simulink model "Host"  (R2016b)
settings: Solver=ode45  StartTime=0.0  StopTime=inf  RelTol=1e-3  AbsTol=1e-6
PreLoadFcn:
  | % load standard fuelsys data
  | load targets_fsysdat;
  | % load standard definitions for the failure signals
  | targets_fsysdat_failsigs;
undefined symbols (not defined in the file or in its folder): period, rep_seq_t, rep_seq_y, serial
libraries: dspnetwork x5, etargetslib x2, instrumentlib x2, demo_controls x1, simulink_extras x1

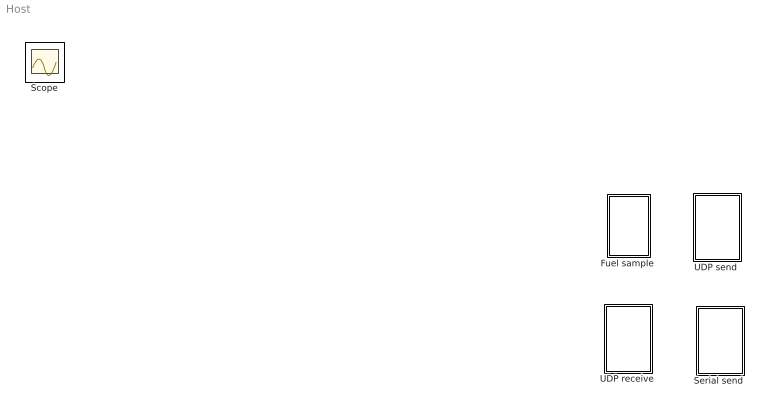
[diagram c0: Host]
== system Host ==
  "Fuel sample " : Subsystem  Commented=on
  "Serial send " : Subsystem  Commented=on
  "UDP receive " : Subsystem
  "UDP send " : Subsystem  Commented=on
  Scope : Scope

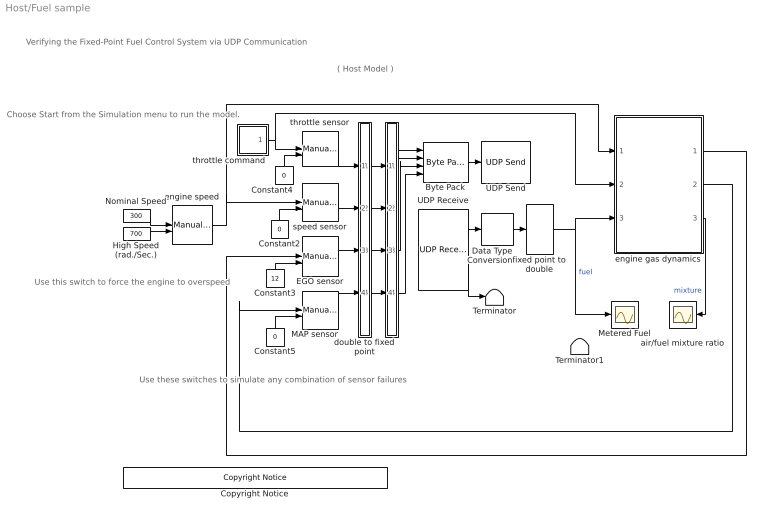
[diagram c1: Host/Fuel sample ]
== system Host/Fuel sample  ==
  note: Use these switches to simulate any combination of sensor failures
  note: Use this switch to force the engine to overspeed
  note: Choose Start from the Simulation menu to run the model.
  note: Verifying the Fixed-Point Fuel Control System via UDP Communication
  note: ( Host Model )
  " " : Subsystem
  Byte Pack : etargetslib/Byte Pack  datatypes={'uint16', 'uint16', 'uint16', 'uint16'}  byteAlign=1
  Constant2 : Constant  Value=0
  Constant3 : Constant  Value=12
  Constant4 : Constant  Value=0
  Constant5 : Constant  Value=0
  Copyright Notice : demo_controls/Copyright Notice  year=2015  prod=idelink
  Data Type Conversion : DataTypeConversion  OutDataTypeStr=fixdt(1,16,8)  ConvertRealWorld=Stored Integer (SI)
  EGO sensor : ManualSwitch
  High Speed (rad./Sec.) : Constant  Value=700
  MAP sensor : ManualSwitch  CurrentSetting=0
  Metered Fuel : Scope
  Nominal Speed : Constant  Value=300
  Terminator : Terminator
  Terminator1 : Terminator
  UDP Receive : dspnetwork/UDP Receive  localURL='0.0.0.0'  localPort=25000  remoteURL='0.0.0.0'  remotePort=-1  recvBufferSize=8192  dims=1  signalDatatype=uint16  isVarSize=off  showBlockingTime=on  blockingTime=1  sampletime=0.01  blockPlatform=HOST
  UDP Send : dspnetwork/UDP Send  remoteURL='255.255.255.255'  remotePort=25555  localURL='255.255.255.255'  localPortSource=Automatically determine  localPort=-1  sampletime=-1  blockPlatform=HOST  separateLengthPort=0
  air/fuel mixture ratio : Scope
  double to fixed point : Subsystem
  engine speed : ManualSwitch
  engine gas dynamics : Subsystem
  fixed point to double : DataTypeConversion  OutDataTypeStr=double  SampleTime=0
  speed sensor : ManualSwitch
  throttle command : Subsystem
  throttle sensor : ManualSwitch
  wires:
  double to fixed point/4(Out4) -> " "/4(In4)
  double to fixed point/1(Out1) -> " "/1(In1)
  double to fixed point/3(Out3) -> " "/3(In3)
  double to fixed point/2(Out2) -> " "/2(In2)
  UDP Receive/2 -> Terminator/1
  Data Type Conversion/1 -> fixed point to double/1
  MAP sensor/1 -> double to fixed point/4(In4)
  engine gas dynamics/3(air/fuel ratio) -> air/fuel mixture ratio/1  "mixture"
  speed sensor/1 -> double to fixed point/2(In2)
  throttle sensor/1 -> double to fixed point/1(In1)
  engine gas dynamics/1(o2_out) -> EGO sensor/1
  engine speed/1 -> engine gas dynamics/1(engine speed), speed sensor/1
  EGO sensor/1 -> double to fixed point/3(In3)
  Constant5/1 -> MAP sensor/2
  Constant3/1 -> EGO sensor/2
  Nominal Speed/1 -> engine speed/1
  Constant4/1 -> throttle sensor/2
  " "/3(Out3) -> Byte Pack/3
  throttle command/1(out_1) -> engine gas dynamics/2(throttle angle), throttle sensor/1
  " "/1(Out1) -> Byte Pack/1
  " "/4(Out4) -> Byte Pack/4
  UDP Receive/1 -> Data Type Conversion/1
  engine gas dynamics/2(MAP) -> MAP sensor/1
  Constant2/1 -> speed sensor/2
  High Speed (rad./Sec.)/1 -> engine speed/2
  fixed point to double/1 -> engine gas dynamics/3(fuel), Metered Fuel/1  "fuel"
  Byte Pack/1 -> UDP Send/1
  " "/2(Out2) -> Byte Pack/2

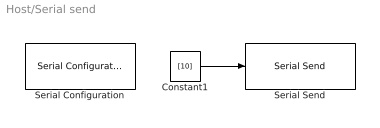
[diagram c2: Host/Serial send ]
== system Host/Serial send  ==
  Constant1 : Constant  Value=[10]  OutDataTypeStr=uint16  SampleTime=0.1
  Serial Configuration : instrumentlib/Serial Configuration  Priority=-200000  ComPortMenu=COM6  ComPort=COM6  ObjConstructor=serial('COM6');  BaudRate=115200  DataBits=8  Parity=none  StopBits=1  FlowControl=none  Timeout=10  ByteOrder=LittleEndian
  Serial Send : instrumentlib/Serial Send  ComPortMenu=COM6  ComPort=COM6  ObjConstructor=serial('COM6');  Header=A  Terminator=B  EnableBlockingMode=off
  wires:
  Constant1/1 -> Serial Send/1

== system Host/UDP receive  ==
  Display : Display
  Terminator1 : Terminator
  UDP Receive2 : dspnetwork/UDP Receive  localURL='0.0.0.0'  localPort=25000  remoteURL='192.128.1.10'  remotePort=-1  recvBufferSize=8192  dims=16  signalDatatype=uint16  isVarSize=off  showBlockingTime=on  blockingTime=1  sampletime=0.01  blockPlatform=HOST
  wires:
  UDP Receive2/1 -> Display/1
  UDP Receive2/2 -> Terminator1/1

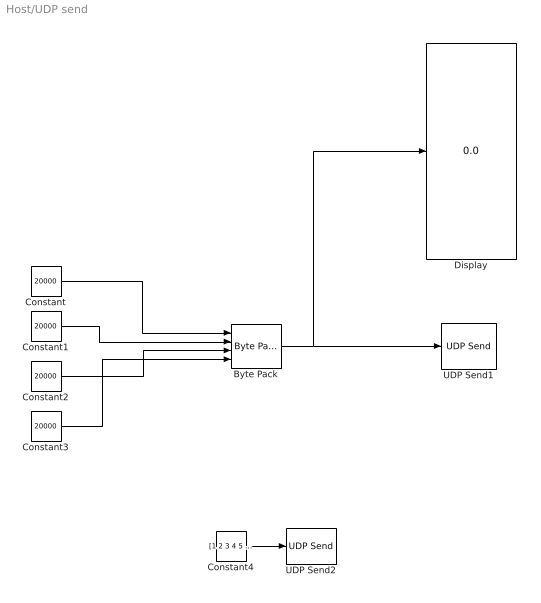
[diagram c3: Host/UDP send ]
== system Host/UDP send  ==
  Byte Pack : etargetslib/Byte Pack  datatypes={'uint16', 'uint16', 'uint16', 'uint16'}  byteAlign=1
  Constant{,1..3} (4 alike) : Constant  Value=20000  OutDataTypeStr=uint16
  Constant4 : Constant  Value=[1 2 3 4 5 6 7 8]  OutDataTypeStr=uint16  SampleTime=0.1
  Display : Display
  UDP Send1 : dspnetwork/UDP Send  remoteURL='192.168.1.10'  remotePort=25555  localURL='255.255.255.255'  localPortSource=Automatically determine  localPort=-1  sampletime=-1  blockPlatform=HOST  separateLengthPort=0
  UDP Send2 : dspnetwork/UDP Send  remoteURL='255.255.255.255'  remotePort=25555  localURL='255.255.255.255'  localPortSource=Automatically determine  localPort=-1  sampletime=-1  blockPlatform=HOST  separateLengthPort=0
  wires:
  Byte Pack/1 -> Display/1, UDP Send1/1
  Constant/1 -> Byte Pack/1
  Constant1/1 -> Byte Pack/2
  Constant2/1 -> Byte Pack/3
  Constant3/1 -> Byte Pack/4
  Constant4/1 -> UDP Send2/1

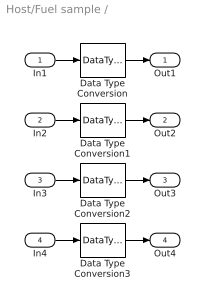
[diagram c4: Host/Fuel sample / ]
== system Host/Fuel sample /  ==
  In1 : Inport
  In2 : Inport  Port=2
  In3 : Inport  Port=3
  In4 : Inport  Port=4
  Data Type Conversion{,1..3} (4 alike) : DataTypeConversion  OutDataTypeStr=uint16  ConvertRealWorld=Stored Integer (SI)
  Out1 : Outport
  Out2 : Outport  Port=2
  Out3 : Outport  Port=3
  Out4 : Outport  Port=4
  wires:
  Data Type Conversion3/1 -> Out4/1
  In4/1 -> Data Type Conversion3/1
  Data Type Conversion2/1 -> Out3/1
  In3/1 -> Data Type Conversion2/1
  Data Type Conversion1/1 -> Out2/1
  In2/1 -> Data Type Conversion1/1
  Data Type Conversion/1 -> Out1/1
  In1/1 -> Data Type Conversion/1

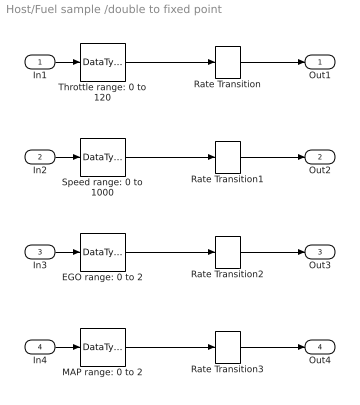
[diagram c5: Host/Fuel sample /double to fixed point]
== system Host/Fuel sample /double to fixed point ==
  In1 : Inport
  In2 : Inport  Port=2
  In3 : Inport  Port=3
  In4 : Inport  Port=4
  EGO range: 0 to 2 : DataTypeConversion  OutDataTypeStr=fixdt(1,16,7)
  MAP range: 0 to 2 : DataTypeConversion  OutDataTypeStr=fixdt(1,16,7)
  Rate Transition{,1..3} (4 alike) : RateTransition  OutPortSampleTime=0.01
  Speed range: 0 to 1000 : DataTypeConversion  OutDataTypeStr=fixdt(1,16,1)
  Throttle range: 0 to 120 : DataTypeConversion  OutDataTypeStr=fixdt(1,16,5)
  Out1 : Outport
  Out2 : Outport  Port=2
  Out3 : Outport  Port=3
  Out4 : Outport  Port=4
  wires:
  In1/1 -> Throttle range: 0 to 120/1
  Throttle range: 0 to 120/1 -> Rate Transition/1
  In2/1 -> Speed range: 0 to 1000/1
  Speed range: 0 to 1000/1 -> Rate Transition1/1
  In3/1 -> EGO range: 0 to 2/1
  EGO range: 0 to 2/1 -> Rate Transition2/1
  In4/1 -> MAP range: 0 to 2/1
  MAP range: 0 to 2/1 -> Rate Transition3/1
  Rate Transition3/1 -> Out4/1
  Rate Transition2/1 -> Out3/1
  Rate Transition1/1 -> Out2/1
  Rate Transition/1 -> Out1/1

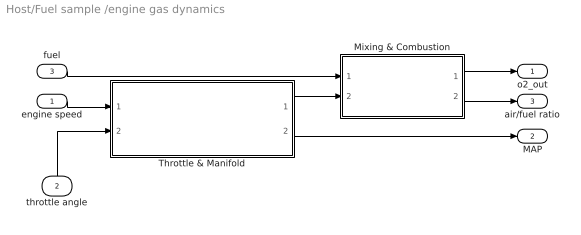
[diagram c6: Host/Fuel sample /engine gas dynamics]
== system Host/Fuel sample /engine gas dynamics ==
  engine speed : Inport
  throttle angle : Inport  Port=2
  fuel : Inport  Port=3
  Mixing & Combustion : Subsystem
  Throttle & Manifold : Subsystem
  o2_out : Outport  InitialOutput=0
  MAP : Outport  Port=2  InitialOutput=0
  air/fuel ratio : Outport  Port=3  InitialOutput=0
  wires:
  Throttle & Manifold/1(Mass Airflow Rate) -> Mixing & Combustion/2(air flow)
  fuel/1 -> Mixing & Combustion/1(fuel rate)
  engine speed/1 -> Throttle & Manifold/1("Engine Speed, N")
  throttle angle/1 -> Throttle & Manifold/2(Throttle Ang.)
  Mixing & Combustion/2(air/fuel ratio) -> air/fuel ratio/1
  Throttle & Manifold/2(MAP (bar)) -> MAP/1
  Mixing & Combustion/1(o2_out) -> o2_out/1

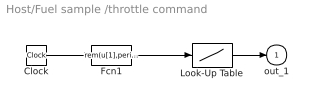
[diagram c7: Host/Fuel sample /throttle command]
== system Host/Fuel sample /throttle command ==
  Clock : Clock
  Fcn1 : Fcn  Expr=rem(u[1],period)
  Look-Up Table : Lookup  InputValues=rep_seq_t  Table=rep_seq_y
  out_1 : Outport  InitialOutput=0
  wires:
  Look-Up Table/1 -> out_1/1
  Clock/1 -> Fcn1/1
  Fcn1/1 -> Look-Up Table/1

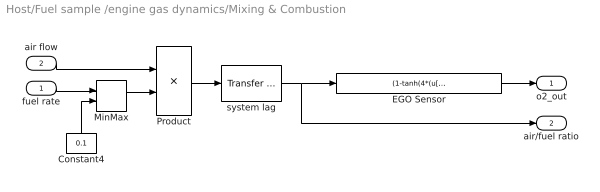
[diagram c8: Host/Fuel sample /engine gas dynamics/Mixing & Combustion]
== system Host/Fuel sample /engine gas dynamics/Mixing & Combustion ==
  fuel rate : Inport
  air flow : Inport  Port=2
  Constant4 : Constant  Value=0.1
  EGO Sensor : Fcn  Expr=(1-tanh(4*(u[1]-14.6)))/2
  MinMax : MinMax  Function=max  Inputs=2
  Product : Product  Inputs=*/
  system lag : simulink_extras/Additional Linear/Transfer Fcn (with initial outputs)  N=3  D=[1 3]  Y0=1/14.6  U0=1/14.6
  o2_out : Outport  InitialOutput=0
  air/fuel ratio : Outport  Port=2  InitialOutput=0
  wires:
  Constant4/1 -> MinMax/2
  fuel rate/1 -> MinMax/1
  MinMax/1 -> Product/2
  Product/1 -> system lag/1
  system lag/1 -> air/fuel ratio/1, EGO Sensor/1
  EGO Sensor/1 -> o2_out/1
  air flow/1 -> Product/1

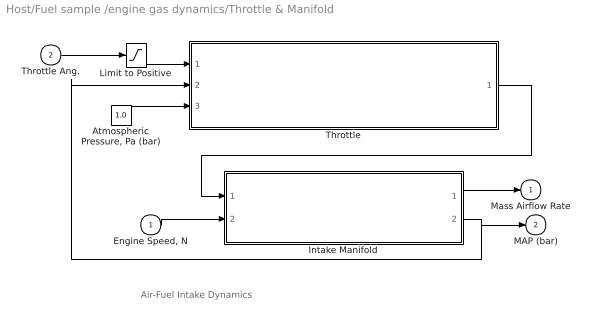
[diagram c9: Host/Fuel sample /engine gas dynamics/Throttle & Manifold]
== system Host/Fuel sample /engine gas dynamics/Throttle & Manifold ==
  note: Air-Fuel Intake Dynamics
  "Engine Speed, N" : Inport
  Throttle Ang. : Inport  Port=2
  "Atmospheric Pressure, Pa (bar)" : Constant  Value=1.0
  Intake Manifold : Subsystem
  Limit to Positive : Saturate  UpperLimit=inf  LowerLimit=0
  Throttle : Subsystem
  Mass Airflow Rate : Outport  InitialOutput=0
  MAP (bar) : Outport  Port=2  InitialOutput=0
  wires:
  Limit to Positive/1 -> Throttle/1("Throttle Angle, theta (deg)")
  Throttle Ang./1 -> Limit to Positive/1
  Throttle/1("Throttle Flow, mdot (g/s)") -> Intake Manifold/1(mdot Input (g/s))
  "Engine Speed, N"/1 -> Intake Manifold/2(N (rad/sec))
  Intake Manifold/1(mdot to Cylinder (g/s)) -> Mass Airflow Rate/1
  "Atmospheric Pressure, Pa (bar)"/1 -> Throttle/3("Atmospheric Pressure, Pa (bar) ")
  Intake Manifold/2("Manifold Pressure, Pm (bar)") -> Throttle/2("Manifold Pressure, Pm (bar)"), MAP (bar)/1

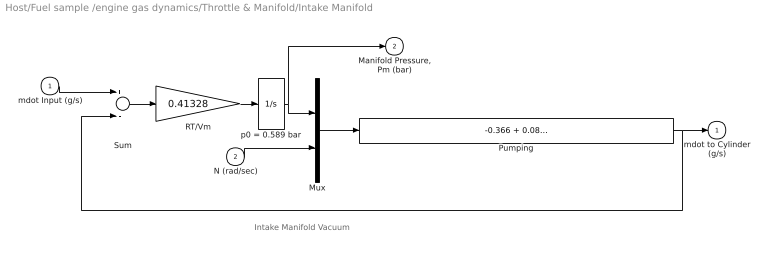
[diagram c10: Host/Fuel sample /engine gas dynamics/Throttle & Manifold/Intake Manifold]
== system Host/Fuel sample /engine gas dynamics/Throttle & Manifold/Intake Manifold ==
  note: Intake Manifold Vacuum
  mdot Input (g/s) : Inport
  N (rad/sec) : Inport  Port=2
  Mux : Mux  Inputs=2
  Pumping : Fcn  Expr=-0.366 + 0.08979*u[1]*u[2] - 0.0337*u[2]*u[1]*u[1] + 0.0001*u[1]*u[2]*u[2]
  RT/Vm : Gain  Gain=0.41328
  Sum : Sum  Inputs=+-
  p0 = 0.589 bar : Integrator  InitialCondition=.589
  mdot to Cylinder (g/s) : Outport  InitialOutput=0
  "Manifold Pressure, Pm (bar)" : Outport  Port=2  InitialOutput=0
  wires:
  mdot Input (g/s)/1 -> Sum/1
  RT/Vm/1 -> p0 = 0.589 bar/1
  N (rad/sec)/1 -> Mux/2
  Mux/1 -> Pumping/1
  p0 = 0.589 bar/1 -> Mux/1, "Manifold Pressure, Pm (bar)"/1
  Sum/1 -> RT/Vm/1
  Pumping/1 -> Sum/2, mdot to Cylinder (g/s)/1

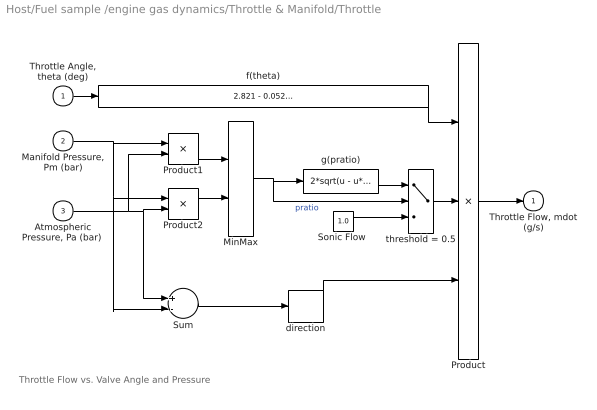
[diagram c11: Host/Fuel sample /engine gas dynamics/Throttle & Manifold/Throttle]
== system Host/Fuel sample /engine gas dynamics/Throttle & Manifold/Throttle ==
  note: Throttle Flow vs. Valve Angle and Pressure
  "Throttle Angle, theta (deg)" : Inport
  "Manifold Pressure, Pm (bar)" : Inport  Port=2
  "Atmospheric Pressure, Pa (bar) " : Inport  Port=3
  MinMax : MinMax  Inputs=2
  Product : Product  Inputs=3
  Product1 : Product  Inputs=*/
  Product2 : Product  Inputs=/*
  "Sonic Flow " : Constant  Value=1.0
  Sum : Sum  Inputs=+-
  direction : Signum
  f(theta) : Fcn  Expr=2.821 - 0.05231*u[1] + 0.10299*u[1]*u[1] - 0.00063*u[1]*u[1]*u[1]
  g(pratio) : Fcn  Expr=2*sqrt(u - u*u)
  threshold = 0.5 : Switch  Threshold=0.5
  "Throttle Flow, mdot (g/s)" : Outport  InitialOutput=0
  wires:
  "Manifold Pressure, Pm (bar)"/1 -> Sum/2, Product2/1, Product1/1
  Product2/1 -> MinMax/2
  Product1/1 -> MinMax/1
  "Atmospheric Pressure, Pa (bar) "/1 -> Sum/1, Product2/2, Product1/2
  g(pratio)/1 -> threshold = 0.5/1
  "Sonic Flow "/1 -> threshold = 0.5/3
  threshold = 0.5/1 -> Product/2
  direction/1 -> Product/3
  Sum/1 -> direction/1
  MinMax/1 -> threshold = 0.5/2, g(pratio)/1  "pratio"
  "Throttle Angle, theta (deg)"/1 -> f(theta)/1
  Product/1 -> "Throttle Flow, mdot (g/s)"/1
  f(theta)/1 -> Product/1
